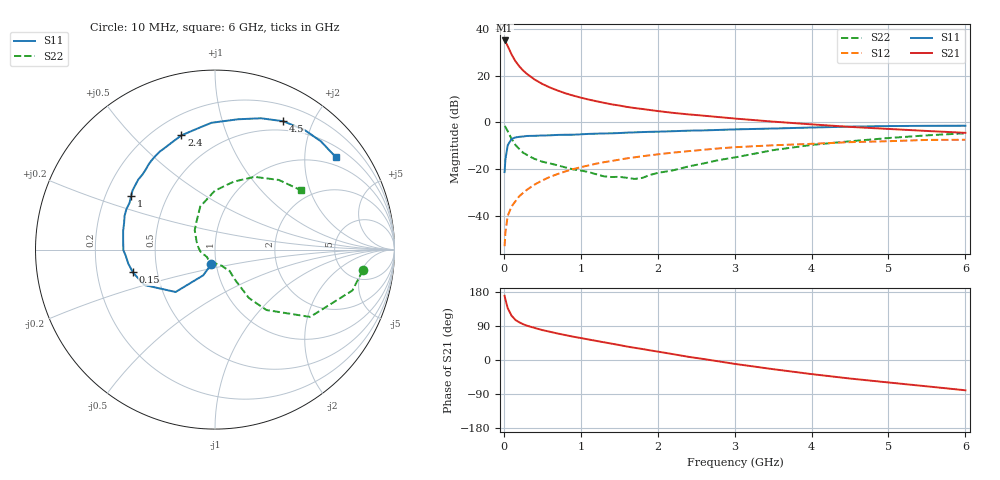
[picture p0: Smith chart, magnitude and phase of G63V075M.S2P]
! SIEMENS Small Signal Semiconductors
! BFG193
! Si NPN RF Bipolar Junction Transistor in SOT223
! VCE = 3 V  IC = 75 mA
! Common Emitter S-Parameters:  August  1996
# GHz  S  MA  R  50
!  f  S11  S21  S12  S22
! GHz  MAG  ANG  MAG  ANG  MAG  ANG  MAG  ANG
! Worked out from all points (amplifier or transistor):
!   36 points, 10 MHz to 6 GHz, reference 50 ohm
!   highest |S21| = 35.2 dB at 10 MHz (marker M1)
!   |S21| within 3 dB of that: start of sweep to 58.44 MHz
!   unconditionally stable (mu >= 1): start of sweep to 13.05 MHz; 243.4 MHz to 2.542 GHz
!   at 250 MHz: K = 1.01, MAG = 25.8 dB, |S12| = -30.3 dB
!   at 1.4 GHz: K = 1.08, MAG = 10.5 dB, |S12| = -16.6 dB
!   at 6 GHz: K = 0.94, MSG = 1.5 dB, |S12| = -7.5 dB
!   S11 on the Smith chart (normalised r, x): 10 MHz: 0.95, -0.16; 150 MHz: 0.36, -0.12; 1 GHz: 0.31, +0.26; 2.4 GHz: 0.31, +0.70; 4.5 GHz: 0.38, +1.60; 6 GHz: 0.75, +2.76
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0.01  0.0856 -104.5  57.33 169.5  0.0022 82.2  0.8319 -8.0
0.02  0.158 -114.7  54.52 160.1  0.0043 74.6  0.7983 -16.6
0.05  0.3225 -132.9  43.49 137.1  0.0098 69.3  0.6491 -35.3
0.1  0.4404 -153.4  28.89 117.1  0.0156 66.8  0.442 -49.6
0.15  0.4749 -164.5  20.62 105.8  0.0202 67.2  0.3292 -55.0
0.2  0.4893 -170.8  16.02 99.5  0.0259 69.7  0.2684 -55.5
0.25  0.4979 -175.8  13.01 94.5  0.0306 70.5  0.2238 -56.1
0.3  0.5106 -179.7  10.98 90.6  0.0357 71.2  0.2004 -56.4
0.4  0.5145 174.1  8.319 84.7  0.0463 70.6  0.1641 -56.0
0.5  0.5225 168.4  6.679 79.0  0.0567 69.9  0.1434 -55.7
0.6  0.5275 163.8  5.599 74.5  0.0677 68.6  0.1312 -57.6
0.7  0.5379 159.5  4.818 69.9  0.0779 67.2  0.1196 -61.0
0.8  0.5424 155.6  4.211 65.7  0.0885 64.9  0.1078 -64.0
1  0.554 147.6  3.396 58.0  0.109 61.6  0.0925 -72.3
1.1  0.5654 144.4  3.097 54.2  0.1189 59.6  0.0859 -80.2
1.6  0.6019 127.9  2.147 35.6  0.1688 48.5  0.0647 -127.1
2.2  0.6458 111.2  1.6 15.4  0.2242 34.5  0.0935 172.8
2.4  0.6634 106.4  1.484 8.4  0.241 30.2  0.1133 155.4
3.5  0.7373 80.0  1.037 -24.2  0.3222 2.5  0.2534 109.0
4.5  0.81 62.0  0.8 -48.9  0.3763 -17.8  0.3928 74.6
5.5  0.8438 45.6  0.654 -69.5  0.4197 -41.5  0.5264 47.5
6  0.8474 37.5  0.596 -79.9  0.4229 -54.9  0.5826 34.5
